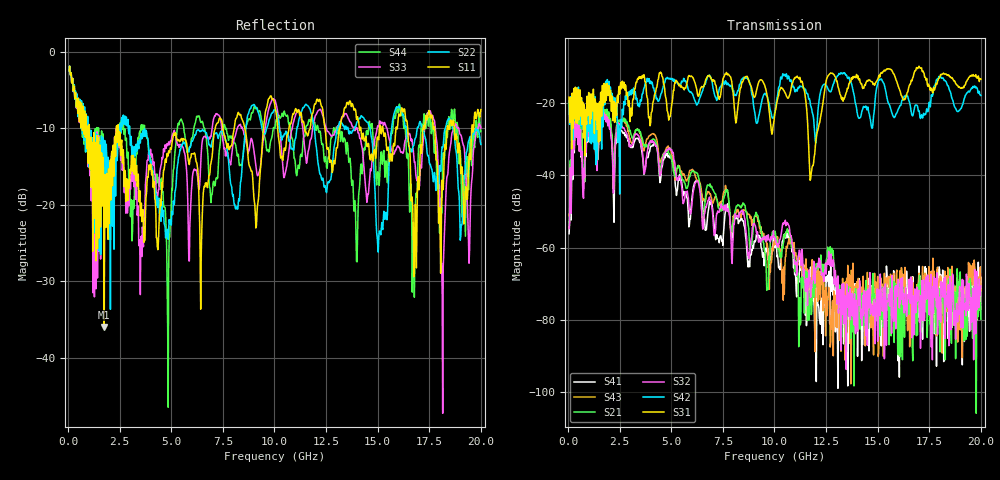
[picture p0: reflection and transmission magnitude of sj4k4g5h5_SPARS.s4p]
! FILE: E:\users\goganessyan\GBX_Backplane\FR408_backplane\1m_OUTBOUND_FEXT\sj4k4g5h5_SPARS.s4p
# MHZ S RI R 50.00
! FREQ  S11  S12  S13  S14
!  S21  S22  S23  S24
!  S31  S32  S33  S34
!  S41  S42  S43  S44
!  REAL  IMAG  REAL  IMAG  REAL  IMAG  REAL  IMAG
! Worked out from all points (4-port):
!   799 points, 50 MHz to 20 GHz, reference 50 ohm
!   strongest paths, dB at 50 MHz, 5.025 GHz, 10.03 GHz, 15.03 GHz, 20 GHz:
!     S31: -18.5, -20.3, -22.6, -13.3, -13.5
!     S42: -19.4, -13.5, -22.3, -14.0, -18.0
!     S32: -54.7, -33.0, -57.3, -71.8, -70.7
!     S21: -53.1, -36.0, -55.5, -82.8, -79.9
!     S43: -50.8, -34.4, -57.1, -90.2, -71.9
!     S41: -56.2, -35.9, -60.0, -73.5, -68.3
!   lowest |S11| = -36.0 dB at 1.75 GHz (marker M1), VSWR 1.03, Z = 48.4 - j0.12 ohm
!   |S11| at or under -10 dB: 1.027 GHz to 2.34 GHz (1.313 GHz wide, 78 % of centre); 2.433 GHz to 7.13 GHz (4.697 GHz wide, 98.2 % of centre); 8.56 GHz to 9.469 GHz (908.8 MHz wide, 10.1 % of centre)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
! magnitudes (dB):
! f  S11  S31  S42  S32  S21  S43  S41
! 50 MHz  -2.5  -18.5  -19.4  -54.7  -53.1  -50.8  -56.2
! 1.75 GHz  -36.0  -14.6  -16.0  -24.4  -23.0  -23.1  -24.3
! 11.15 GHz  -7.6  -13.0  -15.7  -62.6  -67.5  -63.3  -68.7
! 11.78 GHz  -9.0  -39.7  -21.1  -70.4  -78.5  -68.9  -75.5
! 12.9 GHz  -14.6  -12.3  -14.1  -70.2  -64.6  -76.9  -72.2
! 18.12 GHz  -16.8  -12.1  -13.1  -69.9  -74.0  -89.2  -74.3
! 20 GHz  -7.6  -13.5  -18.0  -70.7  -79.9  -71.9  -68.3
